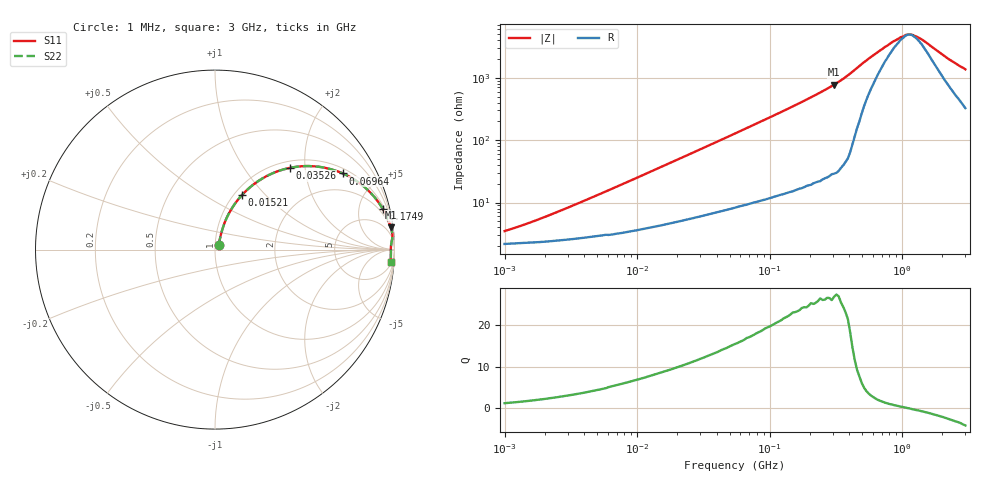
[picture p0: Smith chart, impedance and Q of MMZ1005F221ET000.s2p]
! S-parameter Generated by TDK Corporation
! Copyright(C) 2018 TDK Corporation.
! All Rights Reserved.
! TDK P/N: MMZ1005F221ET000 (Chip Bead)
! Property: |Z|=220¶ at 100MHz
! Size(LxWxT): 1x0.5x0.5mm, 0.039x0.02x0.02inches
! Model Type: s2p (Touchstone File Format Version 1.0)
! Frequency: DC=Yes Start=1MHz Stop=3000MHz 202points Log-sweep
! Model Generated on Aug. 6, 2018
! Port Assignments:
!  1 ---@@@--- 2
! Applicable Conditions:
!  Temperature = 25 degC
!  DC Bias Current = 0 A
!  Small Signal Operation
! Terms and conditions regarding TDK Simulation Models
! (1)This simulation model is being provided solely for informational purposes. Please refer to the specifications of the products in terms of detailed characteristics of such products.
! (2)In no event shall TDK Corporation of any of its subsidiaries be liable for any loss or damage arising, directly or indirectly,
!  From any information contained in this simulation model, including, but not limited to loss or damages arising from any inaccuracies, omissions or errors in connection with such information.
! (3)Any and all copyrights on this simulation model are owned by TDK Corporation.
!  Duplication or redistribution of this simulation model without prior written permission from TDK Corporation is prohibited.
! (4)This simulation model is subject to any modification or change without any prior notice.
! (5)Neither TDK Corporation nor any of its subsidiaries shall make any warranty, express or implied,
!  Including but not limited to the correctness, implied warranties of merchantability and fitness for a particular purpose with respect to this simulation models.
! (6)The use of this simulation model shall be deemed to have consented to the terms and conditions hereof.
# Hz S MA R 50
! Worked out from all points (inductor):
!   201 points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, 1 MHz to 3 GHz, reference 50 ohm
!   read as one part in series: L = 414 nH near 2.947 MHz
!   highest Q = 26.7 at 306.3 MHz (marker M1), where L = 403 nH
!   self-resonance near 1.134 GHz
!   S11 on the Smith chart (normalised r, x): 1 MHz: 1.04, +0.05; 15.21 MHz: 1.09, +0.74; 35.26 MHz: 1.13, +1.66; 69.64 MHz: 1.19, +3.23; 174.9 MHz: 1.34, +8.18; 3 GHz: 8, -27
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1000000  0.03412 50.0  0.9784 -1.5  0.9784 -1.5  0.03412 50.0
1751453  0.05121 61.2  0.9764 -2.6  0.9764 -2.6  0.05121 61.2
3900413  0.1014 69.3  0.9689 -5.6  0.9689 -5.6  0.1014 69.3
8345207  0.2002 69.4  0.9484 -11.4  0.9484 -11.4  0.2002 69.4
1.461624e7  0.3258 64.4  0.9078 -18.9  0.9078 -18.9  0.3258 64.4
1.521322e7  0.3368 63.8  0.9035 -19.5  0.9035 -19.5  0.3368 63.8
2.270269e7  0.4612 57.2  0.8444 -27.3  0.8444 -27.3  0.4612 57.2
3.526298e7  0.6172 47.5  0.7401 -38.0  0.7401 -38.0  0.6172 47.5
5.477226e7  0.7639 36.6  0.5977 -49.7  0.5977 -49.7  0.7639 36.6
6.964249e7  0.829 30.8  0.5128 -55.8  0.5128 -55.8  0.829 30.8
1.081723e8  0.9131 21.4  0.3651 -65.8  0.3651 -65.8  0.9131 21.4
1.748812e8  0.9623 13.6  0.235 -74.0  0.235 -74.0  0.9623 13.6
2.136344e8  0.9738 11.0  0.1917 -76.7  0.1917 -76.7  0.9738 11.0
3.062963e8  0.9871 7.3  0.1272 -80.6  0.1272 -80.6  0.9871 7.3
3.894533e8  0.9916 5.2  0.0907 -82.1  0.0907 -82.1  0.9916 5.2
5.583748e8  0.9858 2.7  0.04866 -71.7  0.04866 -71.7  0.9858 2.7
8.005644e8  0.9805 1.2  0.02827 -45.9  0.02827 -45.9  0.9805 1.2
1.059487e9  0.9803 0.3  0.02021 -12.7  0.02021 -12.7  0.9803 0.3
1.194682e9  0.9802 -0.2  0.02006 9.7  0.02006 9.7  0.9802 -0.2
1.402151e9  0.9802 -0.7  0.02366 32.6  0.02366 32.6  0.9802 -0.7
2.266846e9  0.9807 -2.7  0.04983 65.9  0.04983 65.9  0.9807 -2.7
3e9  0.9804 -4.0  0.07176 72.2  0.07176 72.2  0.9804 -4.0
